PROGRAM TimeSync
VAR
(*
Time format:
FileTime64 		8 Byte len 		begin 1.1.1601	Bit/100ns
DCTime64		8 Byte len		begin 1.1.2000	Bit/100ns
*)
	Test_FileTime64:T_FILETIME64;	// not used only to see where this time begin to see the differnet
	Test_DCTime64:T_DCTIME64;		// not used only to see where this time begin to see the differnet

	
	nLocalTime			: T_FILETIME64;				// Filetime 64 - Local RTOS Time
	nPLC_DC_TASKTime	: T_FILETIME64;				// Filetime 64 - Local DC Time | Local DC Time = System Time see DiffSysTimeToPLCDCTime
	nSysTime AT %I*		: T_FILETIME64;				// Filetime 64 - Sytem Time		
	nExtTime AT %I*		: T_FILETIME64;				// Filetime 64 - TCNet Ext NTP Time
	nSysToExtTimeOffset 	AT %I*	:LINT;			// Offset this is the offset from ExtTime to SysTime
	nSysToExtTimeDeviation 	AT %I*	:LINT;			// Only for Info: Diff from NTP to the NPT Filter time is it < 1ms then is bIsSynchronized = TRUE		
	
	bIsConnected AT %I*:BOOL;			// Connection to the NTP Server
	bIsSynchronized AT %I*:BOOL;		// see nSysToExtTimeDeviation

	FB_LocalSystemTime: FB_LocalSystemTime;		// Functionblock for read the local RTOS Time
	
	dt_LocalTime: DT;			// Time & data - local RTOS Time
	dt_PLC_DC_TASKTime: DT;		// Time & data - This is the time from the TaskInfo Array, this is the same time as the Sytem Time from the NTP Object
	dt_nSysTime: DT;			// Time & data - Sytem Time from the NTP Object
	dt_nExtTime: DT;			// Time & data - NTP Object Ext NTP Time
		
	PlcTaskSystemInfo				: PlcTaskSystemInfo;	// Task Info 
	
	
	DiffSysTimeToPLCDCTime: LINT;			// Local DC Time = System Time
	DiffLocalTimeToExtTime: LINT;			// local Time - ExtTime = same time like the nSysToExtTimeOffset Time
	FB_EcDcTimeCtrl64_1:FB_EcDcTimeCtrl64;	// FB to get Sec/min/Hour... from a DCTime64 
	nExtTime64: ULINT;						// Format DCTime64 from nExtTime
	sec_1: WORD;							// nExtTime Sec
	Min_1: WORD;							// nExtTime Min
	msec_1: WORD;							// nExtTime mSec

	nLocalTimeDC64: ULINT;					// DCtime64 - from local filetime64
	MaxPLCTime: UDINT;


	
	lrTimeoffset: LREAL;				// Offest Time in LREAL [ms] 
	lrTimeDeviation: LREAL;				// Deviation Time [ms] this time show you the diff to the NTP filter time, if its <1ms the is bIsSynchronized = TRUE
	
	FB_CX7000_LED_WD: FB_CX7000_LED_WD;	// NPT Status via WD LED from CX7000

	
END_VAR

PlcTaskSystemInfo:=_TaskInfo[1]; 		// Get Task Info Data we need it to read the PlcTaskSystemInfo.DcTaskTime

dt_PLC_DC_TASKTime:=Systemtime_TO_DT(DCTime64_TO_SYSTEMTIME(LINT_TO_ULINT(PlcTaskSystemInfo.DcTaskTime))); 		// Get Local DC Time to DT
nPLC_DC_TASKTime:=DCTIME64_TO_FILETIME64(LINT_TO_ULINT(PlcTaskSystemInfo.DcTaskTime));							// Get Local DC Time to FileTime64

MaxPLCTime:=MAX(PlcTaskSystemInfo.LastExecTime,MaxPLCTime);


lrTimeoffset:=LINT_TO_LREAL(nSysToExtTimeOffset)/1000/10; // Read NTP Offset Time and convert it to Real in [ms]
lrTimeDeviation:=LINT_TO_LREAL(nSysToExtTimeDeviation)/1000/10; // Read NTP Offset Time and convert it to Real in [ms]


// Read the local time from RTOS
FB_LocalSystemTime(
	sNetID:= , 
	bEnable:=TRUE , 
	dwCycle:= , 
	dwOpt:= , 
	tTimeout:= , 
	bValid=> , 
	systemTime=> , 
	tzID=> );
	
dt_LocalTime:=SystemTime_TO_DT(FB_LocalSystemTime.systemTime);
nLocalTime:=SystemTime_TO_Filetime64(FB_LocalSystemTime.systemTime);

dt_nSysTime:=Filetime64_TO_DT(nSysTime);	// Convert nSysTime to date & time 
dt_nExtTime:=Filetime64_TO_DT(nExtTime);	// Convert nExtTime to date & time 

DiffSysTimeToPLCDCTime:=ULINT_TO_LINT(nPLC_DC_TASKTime-nSysTime);		// Must be 0 because SysTime = Local DC Time
DiffLocalTimeToExtTime:=ULINT_TO_LINT(nExtTime-nPLC_DC_TASKTime);		// Same diff like nSysToExtTimeOffset

// Ext NTP object as trigger for Outputs
nExtTime64:=FILETIME64_TO_DCTIME64(nExtTime);
FB_EcDcTimeCtrl64_1.A_GetMilli (in:=nExtTime64,get=>msec_1); 
FB_EcDcTimeCtrl64_1.A_GetSecond  (in:=nExtTime64,get=>sec_1); 
FB_EcDcTimeCtrl64_1.A_GetMinute   (in:=nExtTime64,get=>Min_1);

// Toggle Outpt every Sec
IF (sec_1 MOD 2) =0 THEN
	gvl.bCX7028_Out_4:=TRUE;
ELSE
	gvl.bCX7028_Out_4:=FALSE;
END_IF


// Set DO NTP Status 
gvl.bCX7028_Out_1:=bIsConnected;
gvl.bCX7028_Out_2:=bIsSynchronized;

// WD LED from CX7000
// Red - no connection
// Green flashing - it is connected to NTP Server but it is not sync (that means that the filter is active and the synchonsation to the NTP Server is running - not with TC!)
// Green on - connection and synchonsation is running
FB_CX7000_LED_WD(
	bEnable:=TRUE , 
	eLED:= , 
	tFlashingTimeP1:= , 
	tFlashingTimeP2:= , 
	bError=> , 
	nErrorID=> );
IF bIsConnected AND NOT bIsSynchronized THEN
	FB_CX7000_LED_WD.eLED :=Tc2_SystemCX.E_CX7000_LED.LED_flashing_GREEN_OFF;
ELSIF bIsConnected AND  bIsSynchronized THEN
	FB_CX7000_LED_WD.eLED :=Tc2_SystemCX.E_CX7000_LED.LED_GREEN ;
ELSE
	FB_CX7000_LED_WD.eLED :=Tc2_SystemCX.E_CX7000_LED.LED_RED ;
END_IF

END_PROGRAM
